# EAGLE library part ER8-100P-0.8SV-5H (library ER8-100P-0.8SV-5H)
Board to Board & Mezzanine Connectors HighSpeed Trans HDR 100P STRGHT 0.76um Source: Datasheet
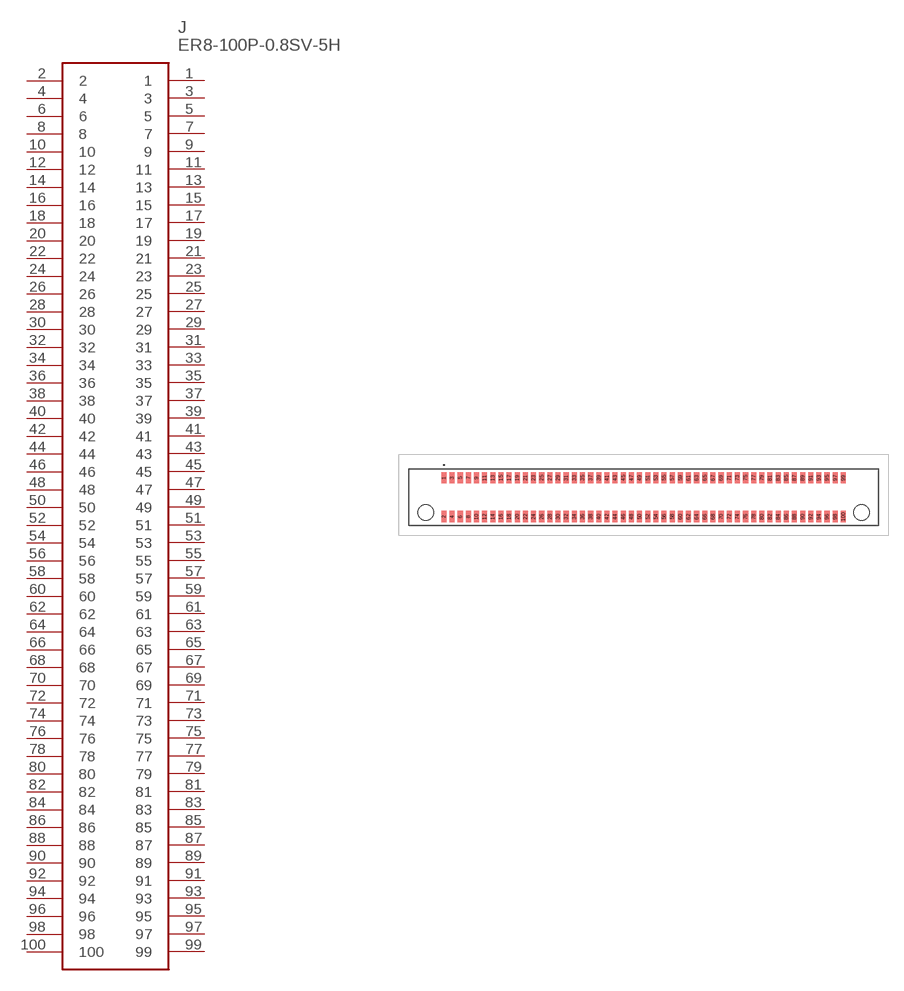
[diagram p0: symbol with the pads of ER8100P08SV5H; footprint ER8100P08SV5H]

Designator prefix J

## ER8-100P-0.8SV-5H (Description: Board to Board & Mezzanine Connectors HighSpeed Trans HDR 100P STRGHT 0.76um; Height: 8.905mm; Manufacturer_Name: Hirose; Manufacturer_Part_Number: ER8-100P-0.8SV-5H; Mouser_Part_Number: 798-ER8-100P-08SV-5H; Mouser_Price-Stock: https://www.mouser.com/Search/Refine.aspx?Keyword=798-ER8-100P-08SV-5H)  [ER8100P08SV5H]
1  1
2  2
3  3
4  4
5  5
6  6
7  7
8  8
9  9
10  10
11  11
12  12
13  13
14  14
15  15
16  16
17  17
18  18
19  19
20  20
21  21
22  22
23  23
24  24
25  25
26  26
27  27
28  28
29  29
30  30
31  31
32  32
33  33
34  34
35  35
36  36
37  37
38  38
39  39
40  40
41  41
42  42
43  43
44  44
45  45
46  46
47  47
48  48
49  49
50  50
51  51
52  52
53  53
54  54
55  55
56  56
57  57
58  58
59  59
60  60
61  61
62  62
63  63
64  64
65  65
66  66
67  67
68  68
69  69
70  70
71  71
72  72
73  73
74  74
75  75
76  76
77  77
78  78
79  79
80  80
81  81
82  82
83  83
84  84
85  85
86  86
87  87
88  88
89  89
90  90
91  91
92  92
93  93
94  94
95  95
96  96
97  97
98  98
99  99
100  100

## Footprint ER8100P08SV5H (pad centres in mm)
ER8-100P-0.8SV-5H-2
smd 0.5 x 1.1: 1 -19.6,1.9; 2 -19.6,-1.9; 3 -18.8,1.9; 4 -18.8,-1.9; 5 -18,1.9; 6 -18,-1.9; 7 -17.2,1.9; 8 -17.2,-1.9; 9 -16.4,1.9; 10 -16.4,-1.9; 11 -15.6,1.9; 12 -15.6,-1.9; 13 -14.8,1.9; 14 -14.8,-1.9; 15 -14,1.9; 16 -14,-1.9; 17 -13.2,1.9; 18 -13.2,-1.9; 19 -12.4,1.9; 20 -12.4,-1.9; 21 -11.6,1.9; 22 -11.6,-1.9; 23 -10.8,1.9; 24 -10.8,-1.9; 25 -10,1.9; 26 -10,-1.9; 27 -9.2,1.9; 28 -9.2,-1.9; 29 -8.4,1.9; 30 -8.4,-1.9; 31 -7.6,1.9; 32 -7.6,-1.9; 33 -6.8,1.9; 34 -6.8,-1.9; 35 -6,1.9; 36 -6,-1.9; 37 -5.2,1.9; 38 -5.2,-1.9; 39 -4.4,1.9; 40 -4.4,-1.9; 41 -3.6,1.9; 42 -3.6,-1.9; 43 -2.8,1.9; 44 -2.8,-1.9; 45 -2,1.9; 46 -2,-1.9; 47 -1.2,1.9; 48 -1.2,-1.9; 49 -0.4,1.9; 50 -0.4,-1.9; 51 0.4,1.9; 52 0.4,-1.9; 53 1.2,1.9; 54 1.2,-1.9; 55 2,1.9; 56 2,-1.9; 57 2.8,1.9; 58 2.8,-1.9; 59 3.6,1.9; 60 3.6,-1.9; 61 4.4,1.9; 62 4.4,-1.9; 63 5.2,1.9; 64 5.2,-1.9; 65 6,1.9; 66 6,-1.9; 67 6.8,1.9; 68 6.8,-1.9; 69 7.6,1.9; 70 7.6,-1.9; 71 8.4,1.9; 72 8.4,-1.9; 73 9.2,1.9; 74 9.2,-1.9; 75 10,1.9; 76 10,-1.9; 77 10.8,1.9; 78 10.8,-1.9; 79 11.6,1.9; 80 11.6,-1.9; 81 12.4,1.9; 82 12.4,-1.9; 83 13.2,1.9; 84 13.2,-1.9; 85 14,1.9; 86 14,-1.9; 87 14.8,1.9; 88 14.8,-1.9; 89 15.6,1.9; 90 15.6,-1.9; 91 16.4,1.9; 92 16.4,-1.9; 93 17.2,1.9; 94 17.2,-1.9; 95 18,1.9; 96 18,-1.9; 97 18.8,1.9; 98 18.8,-1.9; 99 19.6,1.9; 100 19.6,-1.9
hole 1.53 at -21.4,-1.5
hole 1.53 at 21.4,-1.5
